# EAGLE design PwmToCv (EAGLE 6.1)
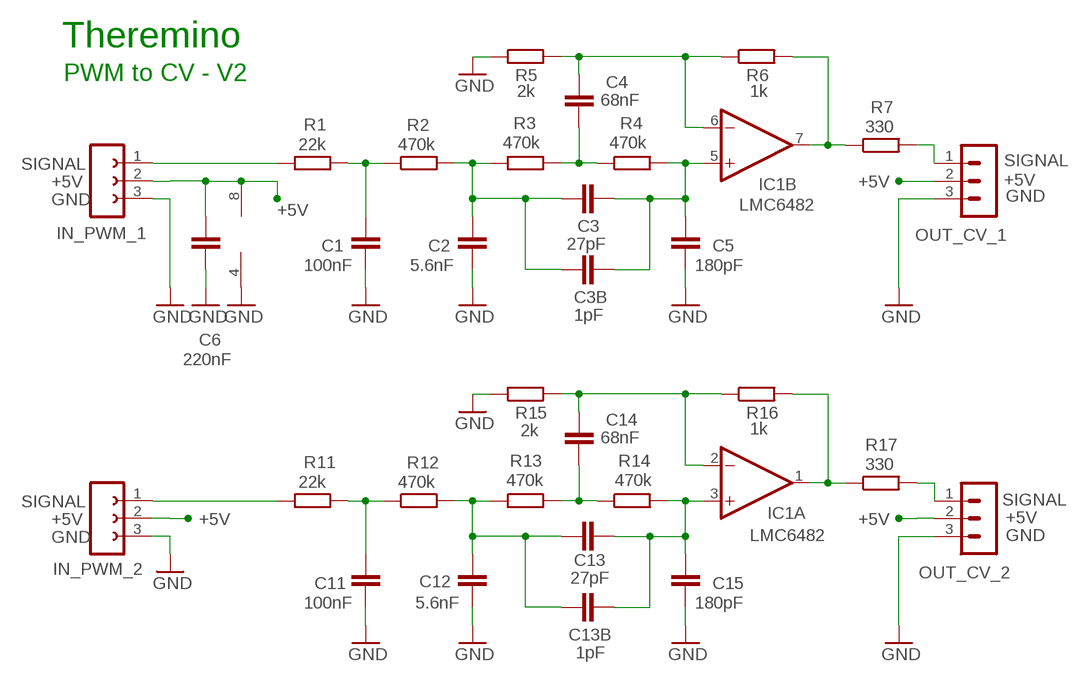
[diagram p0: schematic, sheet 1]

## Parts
C1  100nF  C7.5/3  [C7.5B3]
C2  5.6nF  C5/3  [C5B3]
C3  27pF  C-EU025-024X044  [C025-024X044]
C3B  1pF  C-EU025-024X044  [C025-024X044]
C4  68nF  C7.5/3  [C7.5B3]
C5  180pF  C-EU025-024X044  [C025-024X044]
C6  220nF  C-EU025-024X044  [C025-024X044]
C11  100nF  C7.5/3  [C7.5B3]
C12  5.6nF  C5/3  [C5B3]
C13  27pF  C-EU025-024X044  [C025-024X044]
C13B  1pF  C-EU025-024X044  [C025-024X044]
C14  68nF  C7.5/3  [C7.5B3]
C15  180pF  C-EU025-024X044  [C025-024X044]
IC1  LMC6482  TL072P  [DIL08]
IN_PWM_1  FE03-1"  [FE03-1]
IN_PWM_2  FE03-1"  [FE03-1]
OUT_CV_1  MA03-1L3  [MA03-1_L3]
OUT_CV_2  MA03-1L3  [MA03-1_L3]
R1  22k  R-EU_0204/5  [0204/5]
R2  470k  R-EU_0204/5  [0204/5]
R3  470k  R-EU_0204/5  [0204/5]
R4  470k  R-EU_0204/5  [0204/5]
R5  2k  R-EU_0204/5  [0204/5]
R6  1k  R-EU_0204/5  [0204/5]
R7  330  R-EU_0204/5  [0204/5]
R11  22k  R-EU_0204/5  [0204/5]
R12  470k  R-EU_0204/5  [0204/5]
R13  470k  R-EU_0204/5  [0204/5]
R14  470k  R-EU_0204/5  [0204/5]
R15  2k  R-EU_0204/5  [0204/5]
R16  1k  R-EU_0204/5  [0204/5]
R17  330  R-EU_0204/5  [0204/5]

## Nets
+5V: C6.1 IC1.8(P:V+) IN_PWM_1.2 IN_PWM_2.2 OUT_CV_1.2 OUT_CV_2.2
GND: C1.2 C2.2 C5.2 C6.2 C11.2 C12.2 C15.2 IC1.4(P:V-) IN_PWM_1.3 IN_PWM_2.3 OUT_CV_1.3 OUT_CV_2.3 R5.1 R15.1
N$1: IN_PWM_1.1 R1.2
N$2: C4.1 IC1.6(B:-IN) R5.2 R6.1
N$3: OUT_CV_1.1 R7.2
N$4: C4.2 R3.2 R4.1
N$5: IC1.1(A:OUT) R16.2 R17.1
N$6: C14.1 IC1.2(A:-IN) R15.2 R16.1
N$7: C2.1 C3.1 C3B.1 R2.2 R3.1
N$9: OUT_CV_2.1 R17.2
N$10: C13.2 C13B.2 C15.1 IC1.3(A:+IN) R14.2
N$11: C1.1 R1.1 R2.1
N$12: C14.2 R13.2 R14.1
N$13: C12.1 C13.1 C13B.1 R12.2 R13.1
N$14: C11.1 R11.1 R12.1
N$15: IN_PWM_2.1 R11.2
N$16: C3.2 C3B.2 C5.1 IC1.5(B:+IN) R4.2
N$55: IC1.7(B:OUT) R6.2 R7.1

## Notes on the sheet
- Theremino
- PWM to CV - V2
- SIGNAL | SIGNAL
- +5V | +5V
- GND | GND
- SIGNAL | SIGNAL
- +5V | +5V
- GND | GND

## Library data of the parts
C1 C2 C4 C11 C12 C14 = 00-LIVIO:C: CAPACITOR
C3 C3B C5 C6 C13 C13B C15 = 00-LIVIO:C-EU: CAPACITOR, European symbol
IC1 = linear:TL072: OP AMP
IN_PWM_1 IN_PWM_2 = 02-con-lsta-F:FE03-1: FEMALE HEADER
OUT_CV_1 OUT_CV_2 = 03-con-lstb-M:MA03-1: PIN HEADER
R1-R7 R11-R17 = 00-LIVIO:R-EU_: RESISTOR, European symbol

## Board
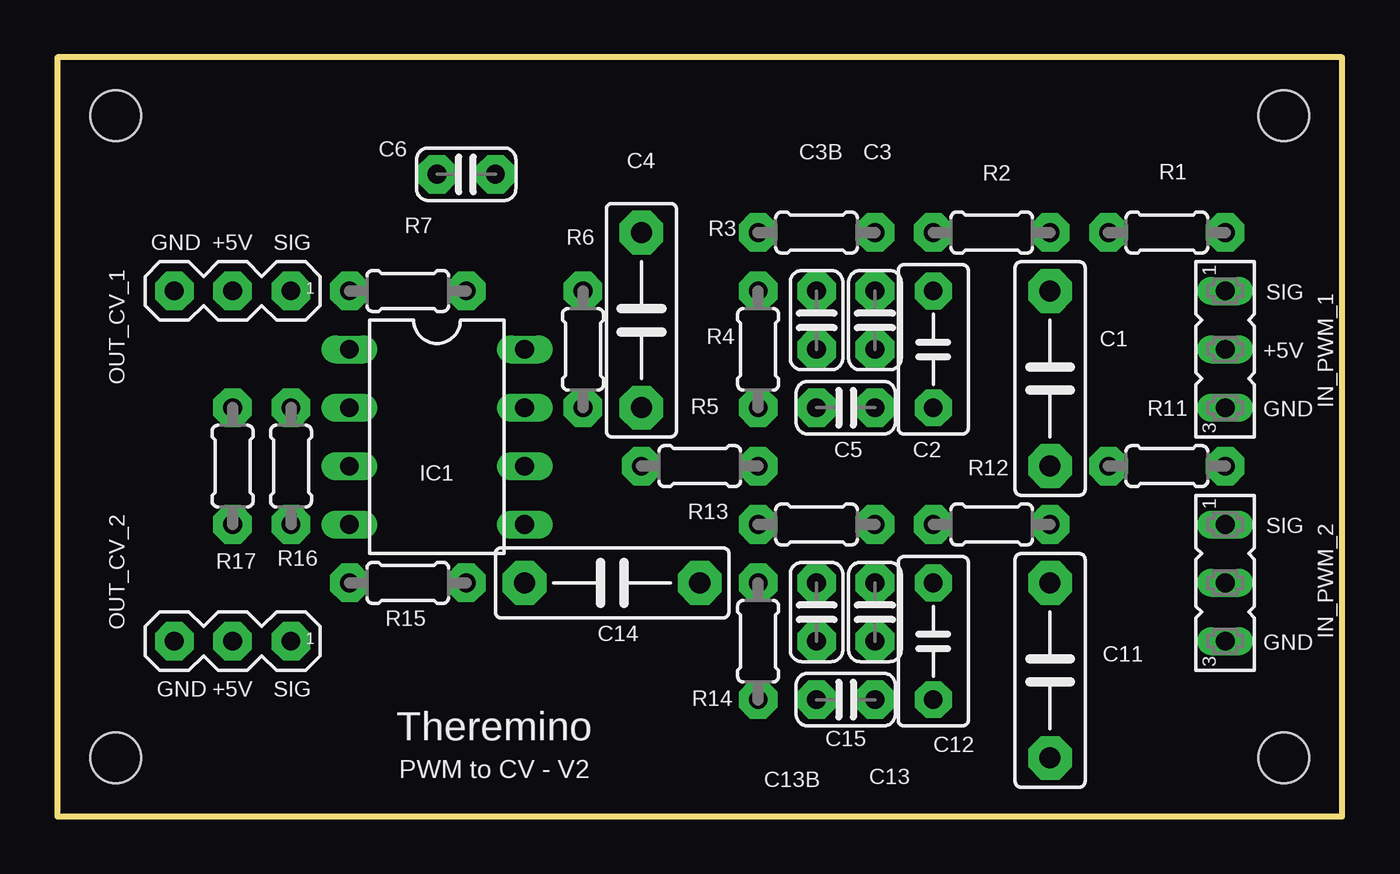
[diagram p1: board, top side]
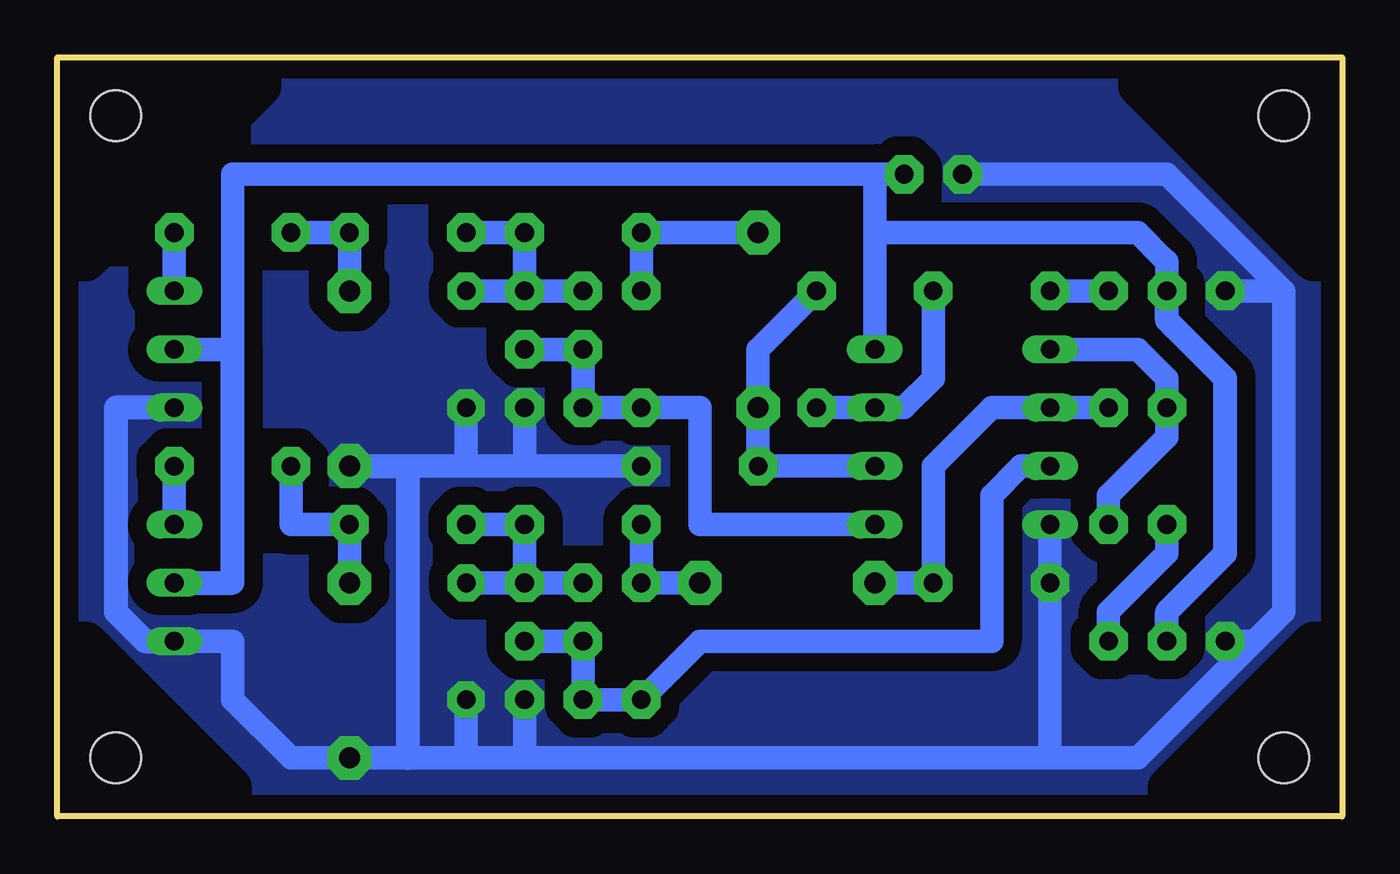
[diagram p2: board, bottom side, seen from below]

Size 55.88 x 33.02 mm. Coordinates in mm from the lower left corner, seen from the top.
Outline: 0,0 55.88,0 55.88,33.02 0,33.02 0,0
Copper layers (1*16): Top 0.035mm / dielectric 1.5mm / Bottom 0.035mm
Design rules: minimum track width 10mil, minimum drill 0.6mm, track to track 8mil, track to pad 8mil, pad to pad 8mil, via to via 8mil, smd to smd 8mil, copper to edge 31mil, drill to drill 8mil, minimum pad ring 5mil, minimum via ring 8mil, stop-mask expansion 4mil, vias tented up to drill 0mil, thermal gap 41mil
Holes 2.2 mm at 53.34,30.48 53.34,2.54 2.54,30.48 2.54,2.54
bRestrict: 4 lines

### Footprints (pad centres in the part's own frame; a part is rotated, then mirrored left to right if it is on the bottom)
C7.5B3 = drill 0.914 pad 1.905 octagon: 1 -3.81,0; 2 3.81,0
C5B3 = drill 0.813 pad 1.6 octagon: 1 -2.54,0; 2 2.54,0
C025-024X044 = drill 0.813 pad 1.676 octagon: 1 -1.27,0; 2 1.27,0
DIL08 = drill 0.813 long: 1 -3.81,-3.81; 2 -1.27,-3.81; 3 1.27,-3.81; 4 3.81,-3.81; 5 3.81,3.81; 6 1.27,3.81; 7 -1.27,3.81; 8 -3.81,3.81
FE03-1 = drill 0.813 long: 1 -2.54,0; 2 0,0; 3 2.54,0
MA03-1_L3 = drill 0.813 pad 1.676 octagon: 1 -2.54,0; 2 0,0; 3 2.54,0
0204/5 = drill 0.813 pad 1.676 octagon: 1 -2.54,0; 2 2.54,0

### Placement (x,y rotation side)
C1  43.18,19.05 270 top
C2  38.1,20.32 270 top
C3  35.56,21.59 270 top
C3B  33.02,21.59 270 top
C4  25.4,21.59 90 top
C5  34.29,17.78 0 top
C6  17.78,27.94 180 top
C11  43.18,6.35 270 top
C12  38.1,7.62 270 top
C13  35.56,8.89 270 top
C13B  33.02,8.89 270 top
C14  24.13,10.16 0 top
C15  34.29,5.08 0 top
IC1  16.51,16.51 270 top
IN_PWM_1  50.8,20.32 270 top
IN_PWM_2  50.8,10.16 270 top
OUT_CV_1  7.62,22.86 180 top
OUT_CV_2  7.62,7.62 180 top
R1  48.26,25.4 0 top
R2  40.64,25.4 180 top
R3  33.02,25.4 180 top
R4  30.48,20.32 270 top
R5  27.94,15.24 180 top
R6  22.86,20.32 270 top
R7  15.24,22.86 180 top
R11  48.26,15.24 0 top
R12  40.64,12.7 180 top
R13  33.02,12.7 180 top
R14  30.48,7.62 270 top
R15  15.24,10.16 0 top
R16  10.16,15.24 270 top
R17  7.62,15.24 270 top

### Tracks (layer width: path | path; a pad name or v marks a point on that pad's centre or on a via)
+5V
  Bottom 1.016: IN_PWM_1.2 48.26,20.32 48.26,27.94 20.32,27.94 | 20.32,27.94 20.32,25.4 | 20.32,25.4 IC1.8 | C6.1 20.32,27.94 | OUT_CV_1.2 7.62,24.13 7.75,24.26 8.89,25.4 20.32,25.4
  Bottom 1.05: OUT_CV_2.2 7.62,8.89 5.08,11.43 5.08,19.05 7.62,21.59 OUT_CV_1.2 | IN_PWM_2.2 48.26,10.16 48.26,20.32
GND
  Bottom 1.016: 45.72,2.54 40.64,2.54 38.1,2.54 | 38.1,2.54 35.56,2.54 | 35.56,2.54 12.7,2.54 | 12.7,2.54 35.56,2.54 | 35.56,2.54 12.7,2.54 | 12.7,2.54 8.89,2.54 3.81,7.62 | 2.54,22.86 7.62,27.94 C6.2 | C11.2 45.72,2.54 | C12.2 38.1,2.54 | C15.2 35.56,2.54 | C1.2 40.64,15.24 38.1,15.24 | 38.1,15.24 C2.2 38.1,15.24 | 38.1,15.24 35.56,15.24 | 35.56,15.24 R5.1 | C5.2 35.56,15.24 | 45.72,2.54 48.26,5.08 48.26,7.62 IN_PWM_2.3 | R15.1 IC1.4 R15.1 | R15.1 12.7,2.54 | 2.54,22.86 OUT_CV_1.3 | 3.81,7.62 OUT_CV_2.3 3.81,7.62 | 3.81,7.62 2.54,8.89 2.54,22.86
  Bottom 1.05: IN_PWM_1.3 53.34,17.78 53.34,8.89 52.07,7.62 IN_PWM_2.3 | C1.2 40.64,15.24 40.64,2.54
  pour Bottom (isolate 0.8, rank 6, no thermals): -1,-1 56.88,-1 56.88,34.02 -1,34.02
N$1
  Bottom 1.016: IN_PWM_1.1 R1.2
N$2
  Bottom 1.016: R6.1 25.4,20.32 C4.1 R5.2 IC1.6
N$3
  Bottom 1.016: OUT_CV_1.1 R7.2
N$4
  Bottom 1.016: C4.2 R3.2 R4.1
N$5
  Bottom 1.016: IC1.1 8.89,20.32 7.62,19.05 R17.1 7.62,16.51 10.16,13.97 R16.2
N$6
  Bottom 1.016: R16.1 11.43,17.78 IC1.2 15.24,17.78 17.78,15.24 R15.2 C14.1
N$7
  Bottom 1.016: R2.2 R3.1 C3.1 | C2.1 C3.1 | C3B.1 C3.1
N$9
  Bottom 1.016: OUT_CV_2.1 10.16,8.89 7.62,11.43 R17.2
N$10
  Bottom 1.016: C13.2 C13B.2 C15.1 R14.2 | IC1.3 13.97,15.24 15.24,13.97 15.24,7.62 27.94,7.62 | 27.94,7.62 R14.2 | R14.2 27.94,7.62 | 27.94,7.62 R14.2
N$11
  Bottom 1.016: C1.1 R2.1 R1.1
N$12
  Bottom 1.016: R13.2 R14.1 | R14.1 C14.2 R14.1
N$13
  Bottom 1.016: R12.2 R13.1 C13.1 | C13.1 C13B.1 | C12.1 C13.1 | C13.1 C13B.1 | C13B.1 C13.1
N$14
  Bottom 1.016: C11.1 R12.1 45.72,12.7 R11.1
N$15
  Bottom 1.016: IN_PWM_2.1 R11.2
N$16
  Bottom 1.016: C3.2 C3B.2 C5.1 R4.2 27.94,17.78 27.94,12.7 IC1.5
N$55
  Bottom 1.016: R7.1 17.78,19.05 19.05,17.78 IC1.7 R6.2

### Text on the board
tNames: GND | +5V | SIG | SIG | +5V | GND | SIG | GND | GND | +5V | SIG | Theremino | PWM to CV - V2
